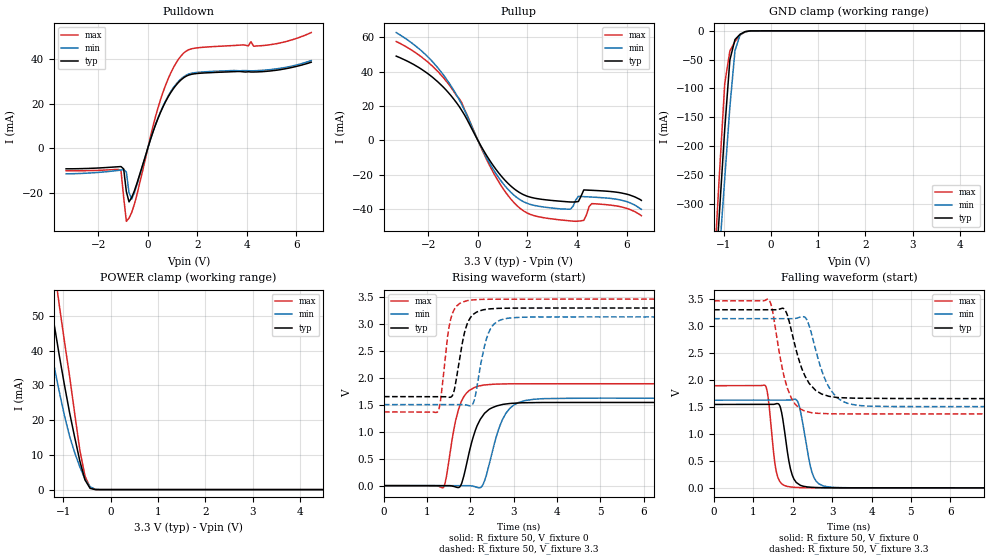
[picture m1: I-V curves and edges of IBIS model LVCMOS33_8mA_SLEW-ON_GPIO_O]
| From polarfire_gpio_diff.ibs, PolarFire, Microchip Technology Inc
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|   Model LVCMOS33_8mA_SLEW-ON_GPIO_O
[Model]   LVCMOS33_8mA_SLEW-ON_GPIO_O
Model_type   Output
Polarity   Non-Inverting
Enable   Active-High
Vmeas =   1.65
Cref =   5p
Rref =   1M
|   typ   min   max
C_comp_pullup   2.605e-12   2.605e-12   2.76e-12
C_comp_pulldown  2.605e-12   2.605e-12   2.76e-12
[Temperature Range]  25C   100C   -40C
[Voltage Range]  3.3   3.135   3.465
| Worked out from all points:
|   slope of the pulldown table from 0 to 0.495 V, typ, clamps not added: 31.7 ohm
|   slope of the pullup table from 0 to 0.495 V, typ, clamps not added: 41.2 ohm
|   GND clamp passes 1 mA (typ) near -0.51 V on its own axis
|   POWER clamp passes 1 mA (typ) near -0.46 V on its own axis
|   rising waveform, R_fixture 50, V_fixture 0: 20-80 % time 346ps typ, 378ps min, 281ps max; typ from 0 V to 1.55 V
|   rising waveform, R_fixture 50, V_fixture 3.3: 20-80 % time 236ps typ, 256ps min, 190ps max; typ from 1.65 V to 3.3 V
|   falling waveform, R_fixture 50, V_fixture 0: 20-80 % time 203ps typ, 246ps min, 161ps max; typ from 1.55 V to 0 V
|   falling waveform, R_fixture 50, V_fixture 3.3: 20-80 % time 432ps typ, 454ps min, 354ps max; typ from 3.3 V to 1.65 V
[GND Clamp]
| Voltage   I(typ)   I(min)   I(max)
-3.3V     -3.213A    -2.957A    -3.541A
-1.191V   -450mA     -505.3mA   -401.1mA
-1.083V   -310.2mA   -380.8mA   -242.7mA
-974.5mV  -170.4mA   -256.4mA   -91.54mA
-866.2mV  -50.48mA   -132.2mA   -34.88mA
-758mV    -15.08mA   -34.24mA   -18.56mA
-649.7mV  -5.883mA   -6.714mA   -7.365mA
-541.4mV  -1.389mA   -1.466mA   -1.709mA
-433.1mV  -123uA     -170uA     -145.5uA
-108.3mV  -6.015nA   -17.98nA   -17.62nA
6.6V      0A         0A         0A
[POWER Clamp]
| Voltage   I(typ)   I(min)   I(max)
-3.3V     320.3mA    266.4mA    379mA
-1.624V   89.11mA    69.3mA     113.8mA
-1.408V   67.23mA    51.37mA    87.82mA
-1.299V   57.08mA    43.14mA    75.67mA
-1.191V   47.51mA    35.38mA    63.94mA
-1.083V   38.51mA    28.09mA    52.96mA
-866.2mV  22.14mA    15.36mA    32.61mA
-649.7mV  8.213mA    6.528mA    11.28mA
-541.4mV  2.791mA    3.019mA    3.88mA
-433.1mV  359.8uA    815.7uA    615.5uA
-216.6mV  159.8nA    4.578uA    2.748uA
6.6V      0A         0A         0A
[Pullup]
| Voltage   I(typ)   I(min)   I(max)
-3.3V     49.01mA    62.7mA     57.5mA
-2.057V   39.19mA    49.12mA    45.97mA
-1.191V   27.78mA    33.97mA    32.88mA
-649.7mV  17.35mA    20.76mA    21.84mA
618.8mV   -14.64mA   -16.83mA   -18.56mA
1.753V    -30.9mA    -34.93mA   -40.07mA
3.733V    -35.78mA   -39.96mA   -46.78mA
4.058V    -35.49mA   -32.52mA   -46.92mA
4.275V    -28.78mA   -32.67mA   -46.46mA
4.599V    -29mA      -32.92mA   -36.72mA
5.79V     -30.53mA   -34.72mA   -38.62mA
6.6V      -34.85mA   -40.05mA   -43.75mA
[Pulldown]
| Voltage   I(typ)   I(min)   I(max)
-3.3V     -9.313mA   -11.56mA   -10.19mA
-1.083V   -8.301mA   -9.851mA   -10.22mA
-974.5mV  -9.371mA   -9.648mA   -22.21mA
-866.2mV  -19.57mA   -10.76mA   -32.96mA
-758mV    -24.21mA   -20.14mA   -31.53mA
-649.7mV  -22.21mA   -22.9mA    -28.95mA
515.6mV   16.17mA    16.44mA    21.91mA
928.1mV   25.06mA    25.48mA    33.89mA
1.444V    31.67mA    32.13mA    42.78mA
4.166V    34.3mA     34.84mA    47.97mA
5.141V    35.03mA    35.65mA    46.96mA
6.6V      38.71mA    39.46mA    52.07mA
[Ramp]
dV/dt_r   0.927346/0.346344n  0.974959/0.377604n  1.1357/0.280507n
dV/dt_f   0.987567/0.432188n  0.977526/0.453646n  1.25749/0.353824n
R_load = 50
[Rising Waveform]
R_fixture = 50
V_fixture = 0
V_fixture_min = 0
V_fixture_max = 0
| Time   V(typ)   V(min)   V(max)
0s        62.35nV    45.17nV    177.2nV
1.37ns    947.1uV    454.8uV    -35.47mV
1.447ns   1.016mV    480.3uV    180.8mV
1.657ns   -25.75mV   550uV      1.21V
1.787ns   25.16mV    593.2uV    1.561V
2.197ns   1.186V     -41.12mV   1.852V
2.319ns   1.337V     74.64mV    1.87V
2.737ns   1.507V     1.224V     1.889V
3.264ns   1.541V     1.581V     1.893V
10ns      1.546V     1.625V     1.893V
[Rising Waveform]
R_fixture = 50
V_fixture = 3.3
V_fixture_min = 3.135
V_fixture_max = 3.465
| Time   V(typ)   V(min)   V(max)
0s        1.654V     1.506V     1.369V
1.249ns   1.654V     1.506V     1.38V
1.309ns   1.654V     1.506V     1.586V
1.471ns   1.645V     1.507V     2.77V
1.558ns   1.651V     1.507V     3.139V
1.926ns   3.007V     1.492V     3.437V
2.099ns   3.202V     1.618V     3.453V
2.42ns    3.282V     2.842V     3.463V
2.763ns   3.296V     3.094V     3.464V
10ns      3.3V       3.135V     3.465V
[Falling Waveform]
R_fixture = 50
V_fixture = 0
V_fixture_min = 0
V_fixture_max = 0
| Time   V(typ)   V(min)   V(max)
0s        1.546V     1.625V     1.893V
1.303ns   1.546V     1.625V     1.893V
1.372ns   1.546V     1.625V     1.686V
1.586ns   1.56V      1.625V     284mV
1.704ns   1.437V     1.625V     87.91mV
1.854ns   713.1mV    1.625V     27.8mV
2.132ns   76.96mV    1.586V     5.709mV
2.488ns   9.81mV     286.1mV    1.084mV
2.759ns   3.097mV    39.97mV    83.56uV
10ns      749.4nV    2.952uV    28.18nV
[Falling Waveform]
R_fixture = 50
V_fixture = 3.3
V_fixture_min = 3.135
V_fixture_max = 3.465
| Time   V(typ)   V(min)   V(max)
0s        3.3V       3.135V     3.465V
1.398ns   3.299V     3.135V     3.481V
1.481ns   3.299V     3.134V     3.298V
1.685ns   3.32V      3.134V     2.388V
1.855ns   3.213V     3.134V     1.86V
2.057ns   2.634V     3.138V     1.551V
2.295ns   2.095V     3.166V     1.425V
2.864ns   1.709V     1.939V     1.373V
3.434ns   1.665V     1.556V     1.369V
10ns      1.654V     1.506V     1.369V
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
